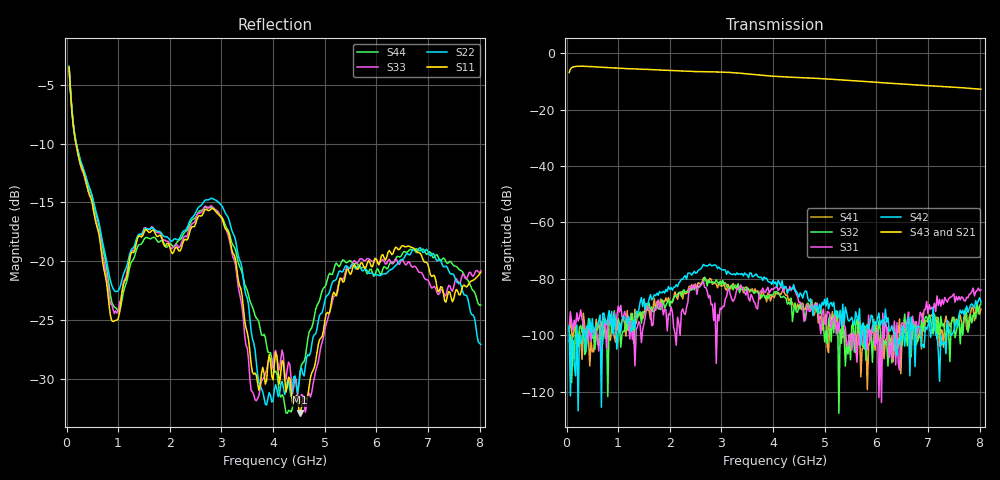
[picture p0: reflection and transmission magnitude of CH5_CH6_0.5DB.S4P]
!Agilent Technologies,E5071C,MY46316741,A.11.02
!Date: Mon Jun 01 10:39:36 2026
!Data & Calibration Information:
!1:CH5 INPUT 2:CH5 OUTPUT 3:CH6 INPUT 4:CH6 OUTPUT
!Freq	S11:SOLT4(ON)	S12:SOLT4(ON)	S13:SOLT4(ON)	S14:SOLT4(ON)
!	S21:SOLT4(ON)	S22:SOLT4(ON)	S23:SOLT4(ON)	S24:SOLT4(ON)
!	S31:SOLT4(ON)	S32:SOLT4(ON)	S33:SOLT4(ON)	S34:SOLT4(ON)
!	S41:SOLT4(ON)	S42:SOLT4(ON)	S43:SOLT4(ON)	S44:SOLT4(ON)
!PortZ  Port1:50+j0  Port2:50+j0  Port3:50+j0  Port4:50+j0
!Above PortZ is port z conversion or system Z0 setting when saving the data.
!When reading, reference impedance value at option line is always used.
# Hz S dB R 50
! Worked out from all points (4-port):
!   320 points, 50 MHz to 8.025 GHz, reference 50 ohm
!   strongest paths, dB at 50 MHz, 2.05 GHz, 4.05 GHz, 6.05 GHz, 8.025 GHz:
!     S43: -6.9, -6.2, -8.3, -10.4, -12.8
!     S21: -7.0, -6.4, -8.5, -10.7, -13.1
!     S42: -96.7, -84.0, -81.1, -92.1, -88.2
!     S31: -97.9, -91.8, -83.0, -122.1, -83.9
!     S32: -102.1, -88.2, -84.6, -94.9, -88.9
!     S41: -98.7, -88.5, -84.9, -100.6, -90.7
!   lowest |S11| = -32.9 dB at 4.525 GHz (marker M1), VSWR 1.05, Z = 49.2 - j2.12 ohm
!   |S11| at or under -10 dB: 184 MHz to end of sweep
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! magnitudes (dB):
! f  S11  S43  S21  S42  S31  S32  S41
! 50 MHz  -3.6  -6.9  -7.0  -96.7  -97.9  -102.1  -98.7
! 875 MHz  -25.0  -5.3  -5.4  -91.6  -94.6  -99.1  -97.0
! 2.825 GHz  -15.5  -6.6  -6.9  -75.4  -89.0  -81.2  -82.0
! 3.85 GHz  -30.4  -8.0  -8.2  -79.8  -84.9  -86.8  -86.2
! 4.525 GHz  -32.9  -8.7  -8.9  -85.0  -88.3  -90.6  -88.8
! 5.425 GHz  -20.7  -9.6  -9.8  -91.9  -103.3  -103.4  -105.6
! 8.025 GHz  -20.9  -12.8  -13.1  -88.2  -83.9  -88.9  -90.7
